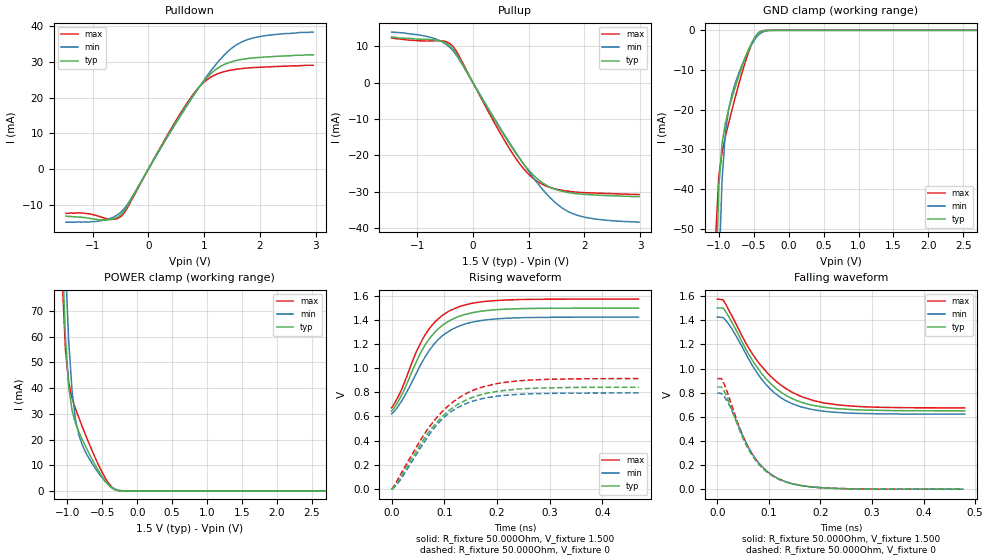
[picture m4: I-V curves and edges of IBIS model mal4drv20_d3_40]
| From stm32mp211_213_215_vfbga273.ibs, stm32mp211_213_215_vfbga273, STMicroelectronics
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[Model] mal4drv20_d3_40
Model_type   I/O
Polarity   Non-Inverting
Enable   Active-High
C_comp   1.836pF   1.830pF   1.844pF
C_comp_pullup   929.639fF   923.197fF   937.397fF
C_comp_pulldown 781.611fF   776.676fF   790.636fF
Vinh = 885.000mV
Vinl = 615.000mV
Vmeas = 750.000mV
Vref = 750.000mV
Rref = 50Ohms
Cref = 0pF
[Model Spec]
Vinh   885.000mV   848.000mV   923.000mV
Vinl   615.000mV   578.000mV   653.000mV
Vmeas   750.000mV   713.000mV   788.000mV
Vref   750.000mV   713.000mV   788.000mV
D_overshoot_ampl_h 0.4 NA   NA
D_overshoot_ampl_l 0.4 NA   NA
D_overshoot_area_l 100.000m NA   NA
D_overshoot_area_h 100.000m NA   NA
[Receiver Thresholds]
Vth = 750.000mV
Vth_min = 713.000mV
Vth_max = 788.000mV
Vinh_ac = 135.000mV
Vinh_dc = 100.000mV
Vinl_ac = -135.000mV
Vinl_dc = -100.000mV
Tslew_ac = 5.000ns
Threshold_sensitivity = 0.5
Reference_supply Pullup_ref
[Temperature Range]   25.000   125.000   -40.000
[Voltage Range]   1.500V   1.425V   1.575V
[GND Clamp Reference]   0.00V   0.00V   0.00V
[C Comp Corner]
| variable   typ   min   max
C_comp 1.844pF   1.836pF   1.830pF
C_comp_pullup 929.639fF   937.397fF   923.197fF
C_comp_pulldown 776.676fF   790.636fF   781.611fF
[Pulldown Reference]   0.00V   0.00V   0.00V
[POWER Clamp Reference]   1.500V   1.425V   1.575V
[Pullup Reference]   1.500V   1.425V   1.575V
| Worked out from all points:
|   slope of the pulldown table from 0 to 0.225 V, typ, clamps not added: 36.8 ohm
|   slope of the pullup table from 0 to 0.225 V, typ, clamps not added: 37.5 ohm
|   GND clamp passes 1 mA (typ) near -0.45 V on its own axis
|   POWER clamp passes 1 mA (typ) near -0.36 V on its own axis
|   rising waveform, R_fixture 50.000Ohm, V_fixture 1.500: 20-80 % time 65.7ps typ, 68.7ps min, 63ps max; typ from 0.645 V to 1.5 V
|   rising waveform, R_fixture 50.000Ohm, V_fixture 0: 20-80 % time 89.8ps typ, 82.9ps min, 95.1ps max; typ from -0.004 V to 0.843 V
|   falling waveform, R_fixture 50.000Ohm, V_fixture 1.500: 20-80 % time 83.5ps typ, 78.4ps min, 92.9ps max; typ from 1.5 V to 0.649 V
|   falling waveform, R_fixture 50.000Ohm, V_fixture 0: 20-80 % time 62.2ps typ, 63.5ps min, 62.2ps max; typ from 0.847 V to 0 V
[GND Clamp]
-1.48V    -1.637A    -1.644A    -1.658A
-1.05V    -67.86mA   -111.2mA   -53.06mA
-1.002V   -39.45mA   -62.21mA   -36.77mA
-954.6mV  -28.48mA   -37.5mA    -30.67mA
-906.8mV  -23.32mA   -25.75mA   -26.73mA
-859.1mV  -19.86mA   -19.72mA   -23.25mA
-763.6mV  -14.17mA   -13.2mA    -16.7mA
-668.2mV  -9.09mA    -8.668mA   -10.65mA
-525mV    -2.932mA   -3.341mA   -3.236mA
-429.5mV  -625.7uA   -1.091mA   -535.7uA
-238.6mV  -2.309uA   -20.7uA    -473nA
2.959V    72.19nA    968.6nA    105nA
[Power Clamp]
-1.459V   654.6mA    675.2mA    655.4mA
-1.077V   94.79mA    129.9mA    83.6mA
-1.03V    59.92mA    88.13mA    55.16mA
-981.8mV  40.46mA    57.96mA    42.01mA
-934.1mV  31.26mA    38.88mA    36.03mA
-886.4mV  26.43mA    28.01mA    32.07mA
-838.6mV  23.06mA    21.89mA    28.58mA
-647.7mV  12.32mA    10.7mA     15.7mA
-504.6mV  5.603mA    5.163mA    7.311mA
-361.4mV  1.062mA    1.366mA    1.412mA
-218.2mV  16.86uA    87.94uA    13.19uA
2.98V     -71.2nA    -1.524uA   -71.42nA
[Pulldown]
-1.48V    -13.2mA    -14.9mA    -12.4mA
-1.193V   -13.5mA    -14.9mA    -12.3mA
-763.6mV  -14.3mA    -14.24mA   -13.85mA
-477.3mV  -12.54mA   -11.85mA   -13.07mA
-334.1mV  -9.268mA   -8.892mA   -9.664mA
286.4mV   7.755mA    7.544mA    8.041mA
668.2mV   17.47mA    17.2mA     17.91mA
906.8mV   22.87mA    22.87mA    22.94mA
1.145V    27.09mA    28.04mA    26mA
1.48V     30.03mA    33.69mA    27.73mA
1.766V    30.96mA    36.21mA    28.32mA
2.959V    32mA       38.4mA     29.1mA
[Pullup]
-1.459V   12.6mA     13.94mA    12.3mA
-743.2mV  11.85mA    12.43mA    11.51mA
-504.6mV  11.05mA    10.81mA    11.4mA
-361.4mV  9.348mA    8.871mA    10.04mA
-265.9mV  7.203mA    6.876mA    7.838mA
688.6mV   -17.61mA   -17.32mA   -18.99mA
927.3mV   -22.74mA   -22.84mA   -24.04mA
1.166V    -26.63mA   -27.85mA   -27.33mA
1.5V      -29.5mA    -33.35mA   -29.38mA
1.786V    -30.47mA   -36.07mA   -30.05mA
2.216V    -30.98mA   -37.62mA   -30.43mA
2.98V     -31.4mA    -38.46mA   -30.84mA
[Ramp]
R_load=50.000Ohm
dV/dt_r   508.170mV/79.000ps  479.578mV/76.000ps  545.010mV/80.000ps
dV/dt_f   508.170mV/73.500ps  479.578mV/72.000ps  545.010mV/78.500ps
[Rising waveform]
R_fixture=50.000Ohm
V_fixture=1.500
V_fixture_min=1.425
V_fixture_max=1.575
0s        645.1mV    621.8mV    671.9mV
14ps      736.8mV    694.4mV    778.1mV
23ps      813.2mV    758.2mV    867.5mV
46ps      1.046V     951.1mV    1.128V
65ps      1.203V     1.105V     1.288V
88ps      1.325V     1.237V     1.409V
121ps     1.418V     1.337V     1.5V
159ps     1.466V     1.389V     1.545V
206ps     1.488V     1.413V     1.565V
469ps     1.5V       1.425V     1.575V
[Rising waveform]
R_fixture=50.000Ohm
V_fixture=0
0s        -3.522mV   -2.041mV   -3.643mV
17ps      94.54mV    76.21mV    118.3mV
55ps      369.2mV    340.5mV    404.3mV
80ps      522.6mV    499.7mV    561mV
97ps      603.1mV    581.9mV    644.4mV
114ps     666mV      642.8mV    711.4mV
152ps     756.1mV    724.4mV    812.4mV
192ps     802.7mV    763.5mV    866.9mV
239ps     827mV      783mV      895.5mV
470ps     842.9mV    795.3mV    914.8mV
[Falling waveform]
R_fixture=50.000Ohm
V_fixture=1.500
V_fixture_min=1.425
V_fixture_max=1.575
0s        1.502V     1.427V     1.576V
11ps      1.502V     1.423V     1.57V
19ps      1.454V     1.386V     1.511V
58ps      1.139V     1.101V     1.19V
94ps      917.3mV    869.8mV    978.1mV
124ps     802.1mV    755.8mV    861mV
162ps     721.8mV    682.7mV    768.8mV
206ps     679.5mV    646.1mV    715.5mV
254ps     660.9mV    631.1mV    690.4mV
480ps     649.3mV    621.9mV    673.5mV
[Falling waveform]
R_fixture=50.000Ohm
V_fixture=0
0s        847.1mV    797.2mV    917mV
8ps       847.1mV    793.4mV    917mV
12ps      821.4mV    775.1mV    883.9mV
24ps      704.1mV    690.3mV    745.1mV
45ps      467.1mV    484.6mV    489.2mV
64ps      302.4mV    319.4mV    316.8mV
88ps      171.5mV    181.3mV    179.4mV
116ps     87.72mV    92.03mV    91.69mV
201ps     11.68mV    12.01mV    12.3mV
477ps     17.28uV    27.2uV     18.25uV
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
